(* Logix 5000 AddOnInstructionDefinition export Banner_IOLM_Param_M_v4; software revision 33.03 *)

TYPE Banner_IOL_Port_v4 :   // UDT that has all of the data items necessary to communicate with a specific Port on a IO-Link Master
STRUCT
   Port_Controlled : INT;   // Each bit represents a port on an IO-Link Master. Set to 1 to tell AOI to control that port.
   Port_Activate : INT;   // Each bit represents a port on an IO-Link Master. When ON that port will process any commands in queue.
   Port_Read : INT;   // Each bit represents a port on an IO-Link Master. Used to determine when device AOI has requested a Read command.
   Port_Write : INT;   // Each bit represents a port on an IO-Link Master. Used to determine when device AOI has requested a Write command.
   Port_RW_Complete : INT;   // Each bit represents a port on an IO-Link Master. Tells device AOI that Read or Write request has been completed.
   Port_Device_Read : INT;
   Data_Transfer : SINT[190];   // Array to transfer data from IO-Master to device AOIs.
END_STRUCT
END_TYPE

TYPE Banner_IOLM_EL_v4 :   // Error Log for Messages to IOLM.
STRUCT
   RW : SINT;   // 0 = Read, 1 = Write, 3 = AOI Failure.
   Port : SINT;   // Port number that generated error.
   Index : INT;   // IO-Link Index for generated error.
END_STRUCT
END_TYPE

TYPE Banner_IOLM_v4 :   // UDT to control IO-Link Masters.
STRUCT
   Message_Source_Data : SINT[190];
   Message_Destination_Data : SINT[190];
   Error_Log : Banner_IOLM_EL_v4[10];
   Error_Write_Retry : BOOL;
   Num_Error_MSGS : DINT;
   IO_Link_Master_Busy : BOOL;   // 0 = While waiting for a command, 1 = Processing command
   AOI_Reset : BOOL;
   Port_Data : Banner_IOL_Port_v4;   // All of the necessary data to work with the various ports of the IO-Link Master.
   Halt_Operation : BOOL;   // When parameter is 1 the AOI is halted as next available time frame.
   AOI_Halted : BOOL;   // AOI is in standby mode until Halt Operation tag is set back to 0.
END_STRUCT
END_TYPE

ADD_ON_INSTRUCTION Banner_IOLM_Param_M_v4   (* revision 4.5, vendor Banner Engineering *)
// AOI that controls an Murr IO-Link Master with Banner devices for parameter data operations.
// Revision note:
// Sub-Index access is now possible for both read and write operations.
VAR_IN_OUT
   Message_Read : MESSAGE; {required}   // Message used to gather data from a device plugged into an Allen Bradley IO-Link Master.
   Message_Write : MESSAGE; {required}   // Message used to send parameter updates to a device plugged into an Allen Bradley IO-Link Master.
   IOLM : Banner_IOLM_v4; {required}
END_VAR
VAR_INPUT
   Type : DINT; {required}   // 0 = CIP Class = 80, 1 = CIP Class = 83. See manual for more information on ISDU format.
END_VAR
VAR
   Lock : DINT; {access None}
   Disable_Timer : BOOL; {access None}
   Byte_Length : SINT; {access None}
   Current_Port : INT; {access None}   // Current port to communicate with via the IO-Link Master.
   Array_Index : DINT; {access None}
   Data_Index : DINT; {access None}
   Message_Timer : TIMER := (PRE := 100); {access None}
   Error_Index : DINT; {access None}
   Message_Timer2 : TIMER := (PRE := 5000); {access None}
   Temp_Index : INT; {access None}
END_VAR

ROUTINE Logic   (* ladder *)
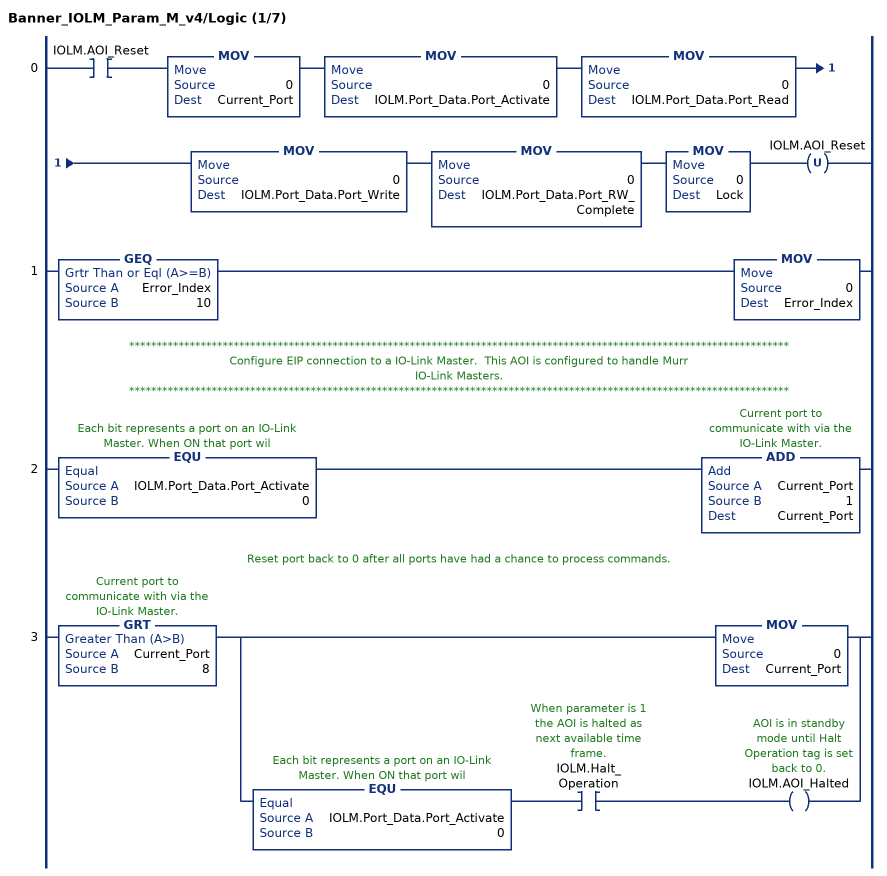
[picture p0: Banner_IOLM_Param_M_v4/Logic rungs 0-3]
   0: XIC(IOLM.AOI_Reset)MOV(0,Current_Port)MOV(0,IOLM.Port_Data.Port_Activate)MOV(0,IOLM.Port_Data.Port_Read)MOV(0,IOLM.Port_Data.Port_Write)MOV(0,IOLM.Port_Data.Port_RW_Complete)MOV(0,Lock)OTU(IOLM.AOI_Reset);
   1: GEQ(Error_Index,10)MOV(0,Error_Index);
   // ************************************************************************************************************************
   // Configure EIP connection to a IO-Link Master.  This AOI is configured to handle Murr
   // IO-Link Masters.
   // ************************************************************************************************************************
   2: EQU(IOLM.Port_Data.Port_Activate,0)ADD(Current_Port,1,Current_Port);
   // Reset port back to 0 after all ports have had a chance to process commands.
   3: GRT(Current_Port,8)[MOV(0,Current_Port) ,EQU(IOLM.Port_Data.Port_Activate,0) XIC(IOLM.Halt_Operation) OTE(IOLM.AOI_Halted) ];
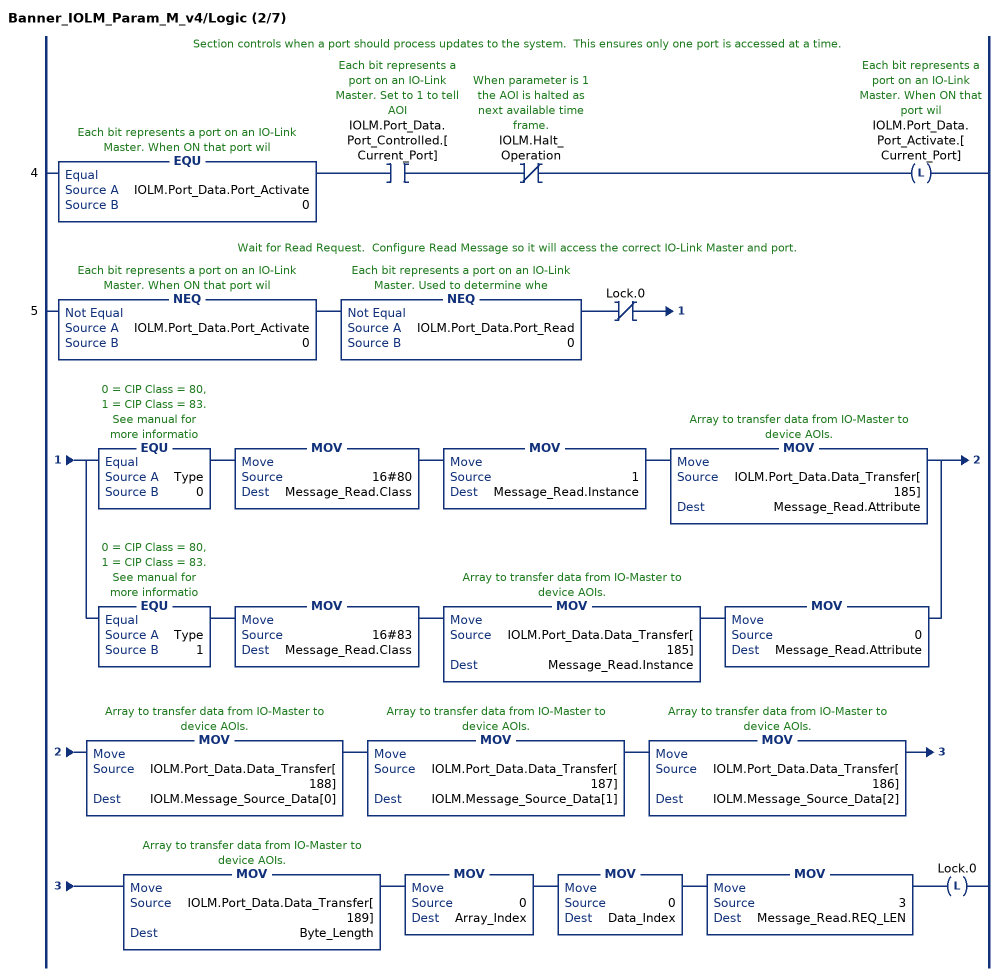
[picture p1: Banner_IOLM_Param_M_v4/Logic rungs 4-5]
   // Section controls when a port should process updates to the system.  This ensures only one port is accessed at a time.
   4: EQU(IOLM.Port_Data.Port_Activate,0)XIC(IOLM.Port_Data.Port_Controlled.[Current_Port])XIO(IOLM.Halt_Operation)OTL(IOLM.Port_Data.Port_Activate.[Current_Port]);
   // Wait for Read Request.  Configure Read Message so it will access the correct IO-Link Master and port.
   5: NEQ(IOLM.Port_Data.Port_Activate,0)NEQ(IOLM.Port_Data.Port_Read,0)XIO(Lock.0)[EQU(Type,0) MOV(16#80,Message_Read.Class) MOV(1,Message_Read.Instance) MOV(IOLM.Port_Data.Data_Transfer[185],Message_Read.Attribute) ,EQU(Type,1) MOV(16#83,Message_Read.Class) MOV(IOLM.Port_Data.Data_Transfer[185],Message_Read.Instance) MOV(0,Message_Read.Attribute) ]MOV(IOLM.Port_Data.Data_Transfer[188],IOLM.Message_Source_Data[0])MOV(IOLM.Port_Data.Data_Transfer[187],IOLM.Message_Source_Data[1])MOV(IOLM.Port_Data.Data_Transfer[186],IOLM.Message_Source_Data[2])MOV(IOLM.Port_Data.Data_Transfer[189],Byte_Length)MOV(0,Array_Index)MOV(0,Data_Index)MOV(3,Message_Read.REQ_LEN)OTL(Lock.0);
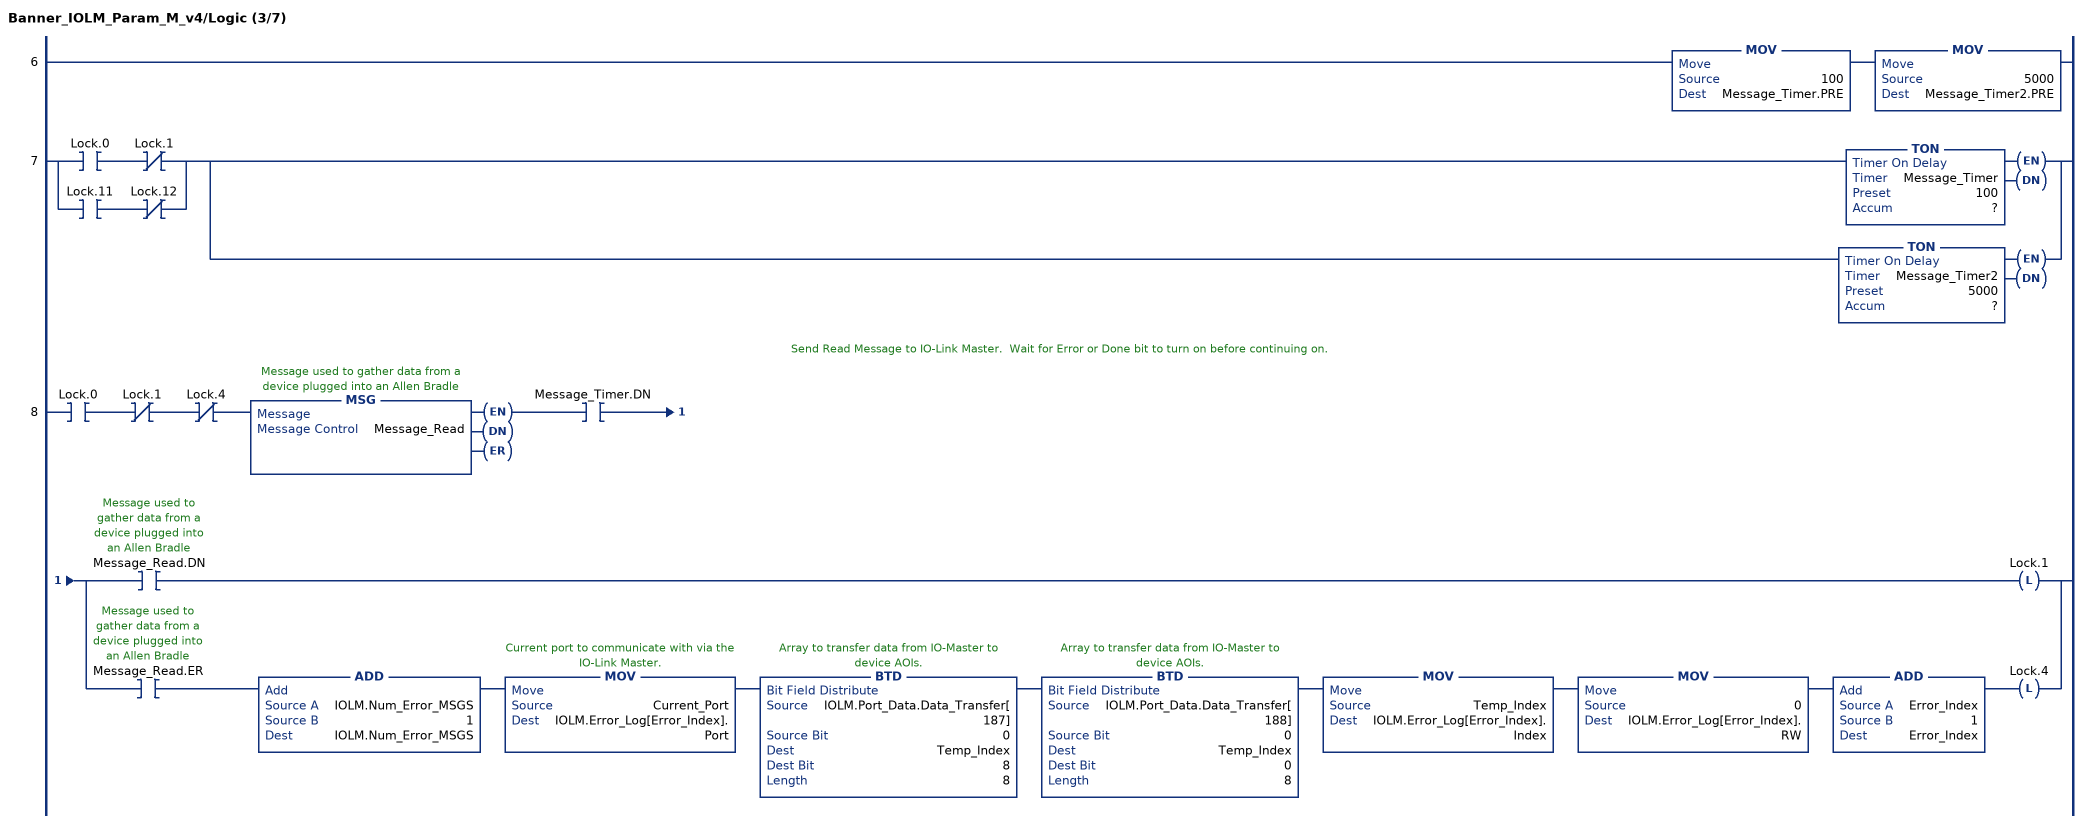
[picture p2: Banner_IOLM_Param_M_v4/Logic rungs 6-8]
   6: MOV(100,Message_Timer.PRE)MOV(5000,Message_Timer2.PRE);
   7: [XIC(Lock.0) XIO(Lock.1) ,XIC(Lock.11) XIO(Lock.12) ][TON(Message_Timer,?,?) ,TON(Message_Timer2,?,?) ];
   // Send Read Message to IO-Link Master.  Wait for Error or Done bit to turn on before continuing on.
   8: XIC(Lock.0)XIO(Lock.1)XIO(Lock.4)MSG(Message_Read)XIC(Message_Timer.DN)[XIC(Message_Read.DN) OTL(Lock.1) ,XIC(Message_Read.ER) ADD(IOLM.Num_Error_MSGS,1,IOLM.Num_Error_MSGS) MOV(Current_Port,IOLM.Error_Log[Error_Index].Port) BTD(IOLM.Port_Data.Data_Transfer[187],0,Temp_Index,8,8) BTD(IOLM.Port_Data.Data_Transfer[188],0,Temp_Index,0,8) MOV(Temp_Index,IOLM.Error_Log[Error_Index].Index) MOV(0,IOLM.Error_Log[Error_Index].RW) ADD(Error_Index,1,Error_Index) OTL(Lock.4) ];
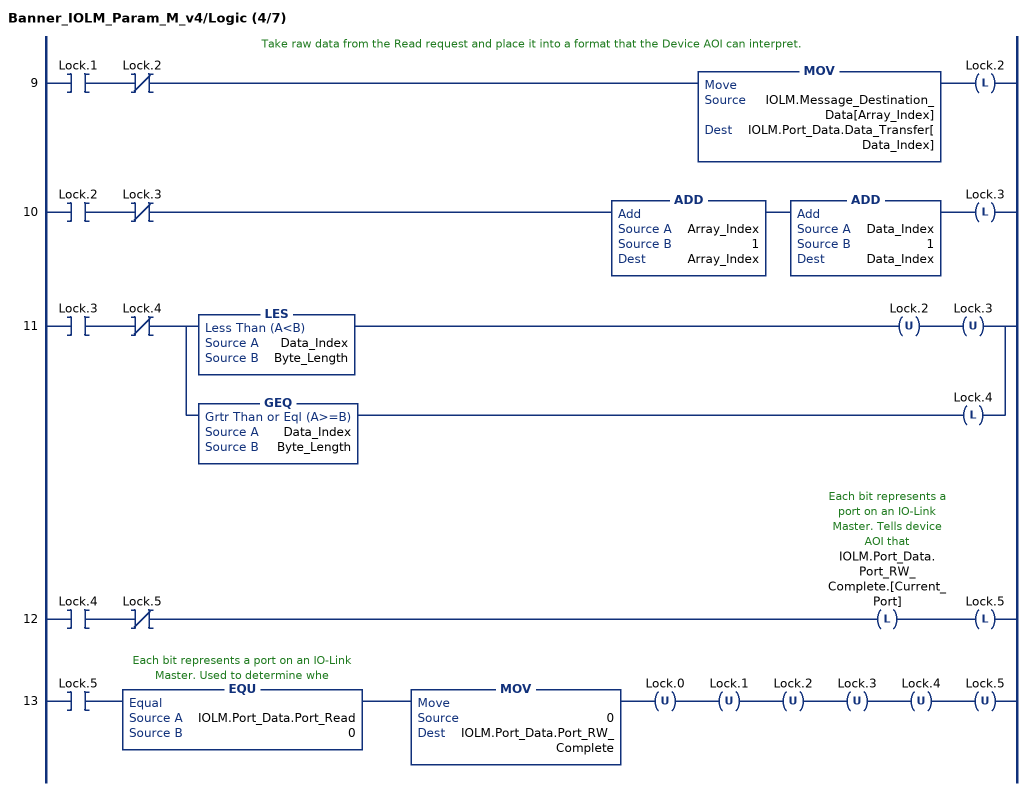
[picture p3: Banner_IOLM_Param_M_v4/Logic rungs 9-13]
   // Take raw data from the Read request and place it into a format that the Device AOI can interpret.
   9: XIC(Lock.1)XIO(Lock.2)MOV(IOLM.Message_Destination_Data[Array_Index],IOLM.Port_Data.Data_Transfer[Data_Index])OTL(Lock.2);
   10: XIC(Lock.2)XIO(Lock.3)ADD(Array_Index,1,Array_Index)ADD(Data_Index,1,Data_Index)OTL(Lock.3);
   11: XIC(Lock.3)XIO(Lock.4)[LES(Data_Index,Byte_Length) OTU(Lock.2) OTU(Lock.3) ,GEQ(Data_Index,Byte_Length) OTL(Lock.4) ];
   12: XIC(Lock.4)XIO(Lock.5)OTL(IOLM.Port_Data.Port_RW_Complete.[Current_Port])OTL(Lock.5);
   13: XIC(Lock.5)EQU(IOLM.Port_Data.Port_Read,0)MOV(0,IOLM.Port_Data.Port_RW_Complete)OTU(Lock.0)OTU(Lock.1)OTU(Lock.2)OTU(Lock.3)OTU(Lock.4)OTU(Lock.5);
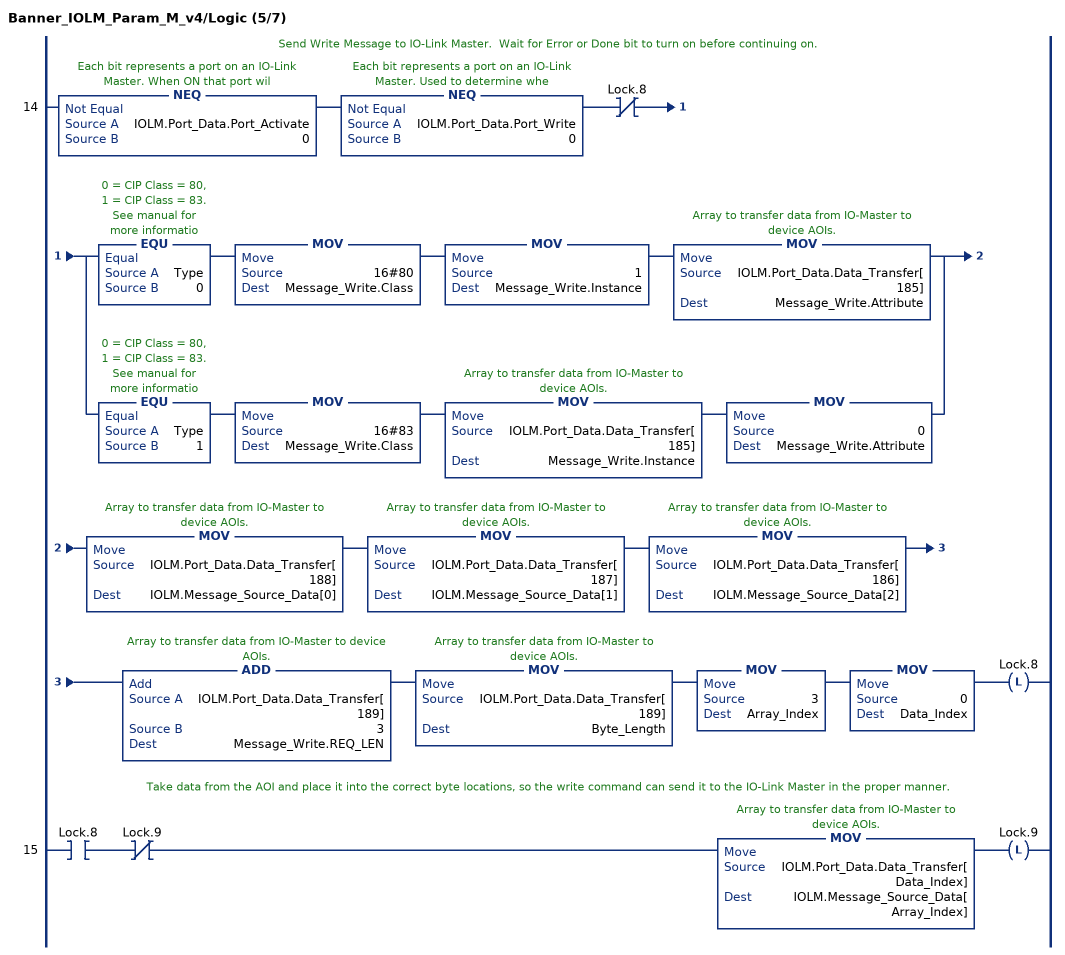
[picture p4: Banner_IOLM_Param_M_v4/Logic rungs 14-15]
   // Send Write Message to IO-Link Master.  Wait for Error or Done bit to turn on before continuing on.
   14: NEQ(IOLM.Port_Data.Port_Activate,0)NEQ(IOLM.Port_Data.Port_Write,0)XIO(Lock.8)[EQU(Type,0) MOV(16#80,Message_Write.Class) MOV(1,Message_Write.Instance) MOV(IOLM.Port_Data.Data_Transfer[185],Message_Write.Attribute) ,EQU(Type,1) MOV(16#83,Message_Write.Class) MOV(IOLM.Port_Data.Data_Transfer[185],Message_Write.Instance) MOV(0,Message_Write.Attribute) ]MOV(IOLM.Port_Data.Data_Transfer[188],IOLM.Message_Source_Data[0])MOV(IOLM.Port_Data.Data_Transfer[187],IOLM.Message_Source_Data[1])MOV(IOLM.Port_Data.Data_Transfer[186],IOLM.Message_Source_Data[2])ADD(IOLM.Port_Data.Data_Transfer[189],3,Message_Write.REQ_LEN)MOV(IOLM.Port_Data.Data_Transfer[189],Byte_Length)MOV(3,Array_Index)MOV(0,Data_Index)OTL(Lock.8);
   // Take data from the AOI and place it into the correct byte locations, so the write command can send it to the IO-Link Master in the proper manner.
   15: XIC(Lock.8)XIO(Lock.9)MOV(IOLM.Port_Data.Data_Transfer[Data_Index],IOLM.Message_Source_Data[Array_Index])OTL(Lock.9);
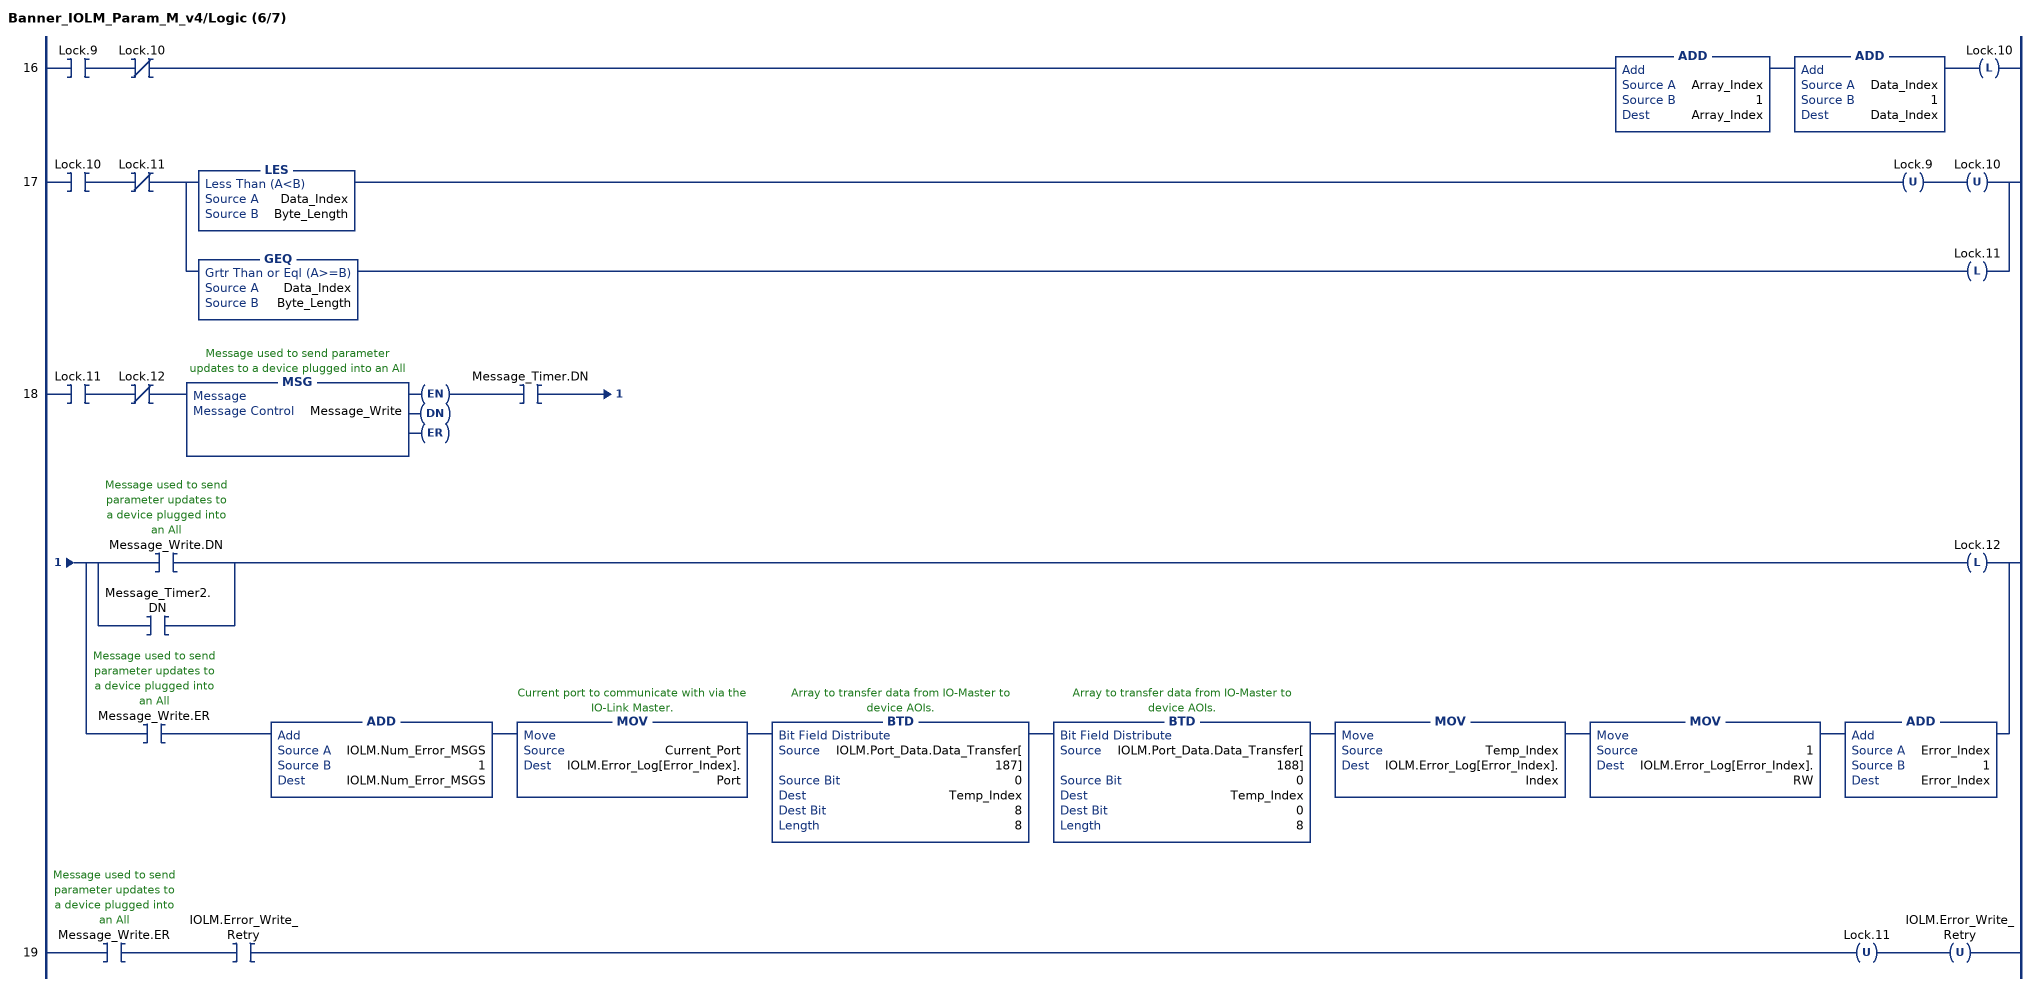
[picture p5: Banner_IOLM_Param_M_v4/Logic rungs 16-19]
   16: XIC(Lock.9)XIO(Lock.10)ADD(Array_Index,1,Array_Index)ADD(Data_Index,1,Data_Index)OTL(Lock.10);
   17: XIC(Lock.10)XIO(Lock.11)[LES(Data_Index,Byte_Length) OTU(Lock.9) OTU(Lock.10) ,GEQ(Data_Index,Byte_Length) OTL(Lock.11) ];
   18: XIC(Lock.11)XIO(Lock.12)MSG(Message_Write)XIC(Message_Timer.DN)[[XIC(Message_Write.DN) ,XIC(Message_Timer2.DN) ] OTL(Lock.12) ,XIC(Message_Write.ER) ADD(IOLM.Num_Error_MSGS,1,IOLM.Num_Error_MSGS) MOV(Current_Port,IOLM.Error_Log[Error_Index].Port) BTD(IOLM.Port_Data.Data_Transfer[187],0,Temp_Index,8,8) BTD(IOLM.Port_Data.Data_Transfer[188],0,Temp_Index,0,8) MOV(Temp_Index,IOLM.Error_Log[Error_Index].Index) MOV(1,IOLM.Error_Log[Error_Index].RW) ADD(Error_Index,1,Error_Index) ];
   19: XIC(Message_Write.ER)XIC(IOLM.Error_Write_Retry)OTU(Lock.11)OTU(IOLM.Error_Write_Retry);
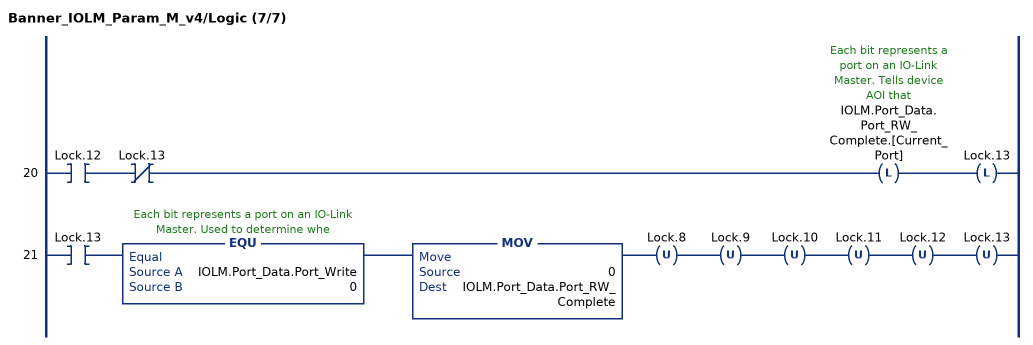
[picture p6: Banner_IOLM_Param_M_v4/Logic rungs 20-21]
   20: XIC(Lock.12)XIO(Lock.13)OTL(IOLM.Port_Data.Port_RW_Complete.[Current_Port])OTL(Lock.13);
   21: XIC(Lock.13)EQU(IOLM.Port_Data.Port_Write,0)MOV(0,IOLM.Port_Data.Port_RW_Complete)OTU(Lock.8)OTU(Lock.9)OTU(Lock.10)OTU(Lock.11)OTU(Lock.12)OTU(Lock.13);
END_ROUTINE
END_ADD_ON_INSTRUCTION
